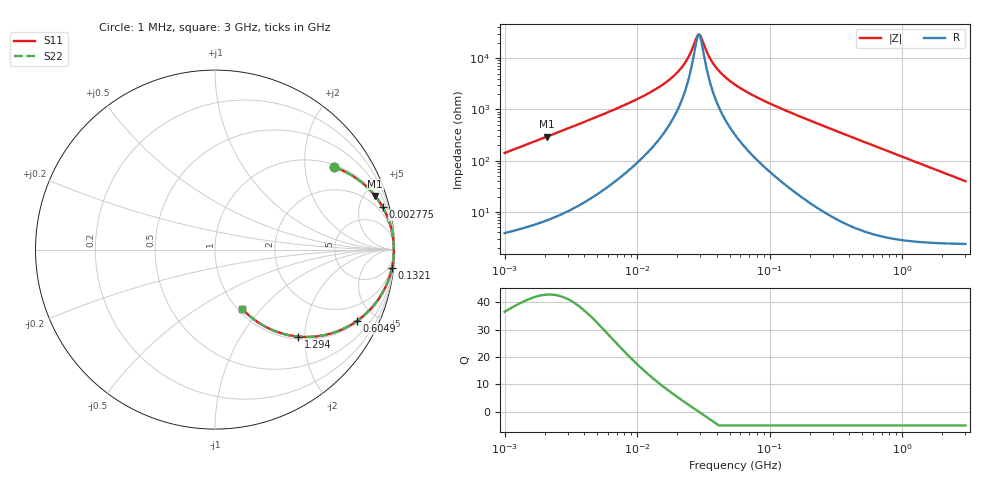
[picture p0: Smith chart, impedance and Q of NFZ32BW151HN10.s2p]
! NFZ32BW151HN10
# Hz S RI R 50
!Freq.(Hz) S11(Real) S11(Imag) S21(Real) S21(Imag) S12(Real) S12(Imag) S22(Real) S22(Imag)
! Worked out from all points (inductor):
!   401 points, 1 MHz to 3 GHz, reference 50 ohm
!   read as one part in series: L = 22.4 uH near 1.041 MHz
!   highest Q = 42.8 at 2.097 MHz (marker M1), where L = 22.5 uH
!   self-resonance near 28.87 MHz
!   S11 on the Smith chart (normalised r, x): 1 MHz: 1.08, +2.83; 2.775 MHz: 1.19, +7.85; 132.1 MHz: 2, -19; 604.9 MHz: 1.07, -3.96; 1.294 GHz: 1.05, -1.85; 3 GHz: 1.05, -0.80
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1000000  0.6625 0.4594  0.3375 -0.4594  0.3375 -0.4594  0.6625 0.4594
2097170  0.892 0.299  0.108 -0.299  0.108 -0.299  0.892 0.299
2775447  0.9341 0.2364  0.0659 -0.2364  0.0659 -0.2364  0.9341 0.2364
3823119  0.963 0.1759  0.037 -0.1759  0.037 -0.1759  0.963 0.1759
8686058  0.9908 0.074  0.00921 -0.074  0.00921 -0.074  0.9908 0.074
1.461624e7  0.9952 0.0364  0.00483 -0.0364  0.00483 -0.0364  0.9952 0.0364
1.821614e7  0.996 0.0238  0.00403 -0.0238  0.00403 -0.0238  0.996 0.0238
2.181181e7  0.9963 0.0144  0.00366 -0.0144  0.00366 -0.0144  0.9963 0.0144
2.459509e7  0.9965 0.00843  0.00351 -0.00843  0.00351 -0.00843  0.9965 0.00843
2.829425e7  0.9966 0.00159  0.00344 -0.00159  0.00344 -0.00159  0.9966 0.00159
2.944989e7  0.9966 -0.000354  0.00343 0.000354  0.00343 0.000354  0.9966 -0.000354
3.820236e7  0.9964 -0.0131  0.00361 0.0131  0.00361 0.0131  0.9964 -0.0131
4.483659e7  0.9961 -0.0214  0.0039 0.0214  0.0039 0.0214  0.9961 -0.0214
5.477226e7  0.9955 -0.0325  0.00451 0.0325  0.00451 0.0325  0.9955 -0.0325
1.321429e8  0.9855 -0.1032  0.0145 0.1032  0.0145 0.1032  0.9855 -0.1032
2.094008e8  0.9676 -0.1654  0.0324 0.1654  0.0324 0.1654  0.9676 -0.1654
3.741707e8  0.9076 -0.2806  0.0924 0.2806  0.0924 0.2806  0.9076 -0.2806
6.049187e8  0.7927 -0.3962  0.2073 0.3962  0.2073 0.3962  0.7927 -0.3962
8.005644e8  0.6876 -0.4532  0.3124 0.4532  0.3124 0.4532  0.6876 -0.4532
1.294266e9  0.4621 -0.4846  0.5379 0.4846  0.5379 0.4846  0.4621 -0.4846
2.01032e9  0.2701 -0.4239  0.7299 0.4239  0.7299 0.4239  0.2701 -0.4239
3e9  0.1519 -0.3302  0.8481 0.3302  0.8481 0.3302  0.1519 -0.3302
